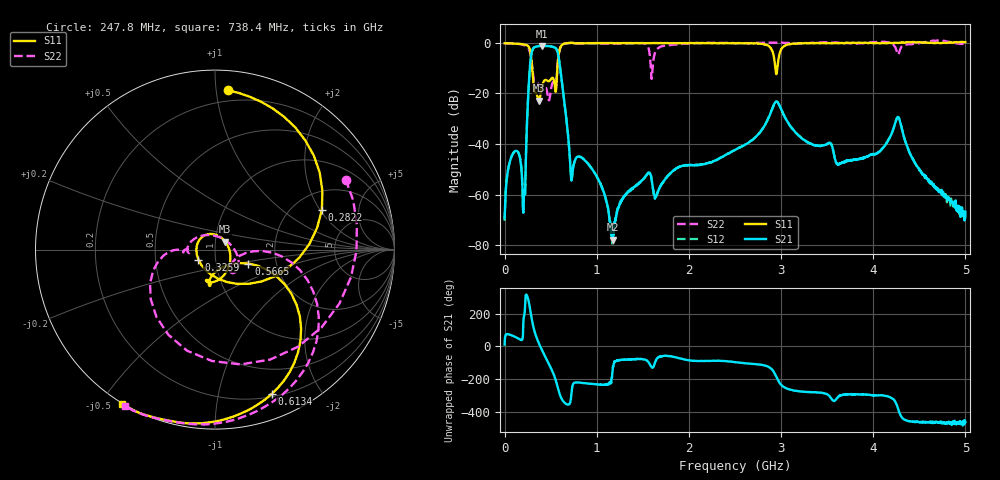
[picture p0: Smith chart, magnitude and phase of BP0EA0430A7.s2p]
!Agilent Technologies,E8358A,US41080443,A.07.50.56
!Agilent E8358A: A.07.50.56
!Date: Friday, November 10, 2017 09:13:59
!Correction: S11(Full 2 Port(1,2))
!S21(Full 2 Port(1,2))
!S12(Full 2 Port(1,2))
!S22(Full 2 Port(1,2))
!S2P File: Measurements: S11, S21, S12, S22:
# Hz S  dB  R 50
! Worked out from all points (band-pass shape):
!   1601 points, 1 MHz to 5 GHz, reference 50 ohm
!   highest |S21| = -1.17 dB at 410.3 MHz (marker M1); lowest = -77.8 dB at 1.173 GHz (marker M2)
!   |S21| within 3 dB of the highest: 292.9 MHz to 579.1 MHz (286.2 MHz wide, 65.7 % of centre)
!   lowest |S11| = -22.8 dB at 372.8 MHz (marker M3), VSWR 1.16, Z = 55.9 + j4.98 ohm
!   |S11| at or under -10 dB: 300.8 MHz to 573.1 MHz (272.3 MHz wide, 62.3 % of centre); 2.939 GHz to 2.96 GHz (21.16 MHz wide, 0.718 % of centre)
!   |S22| runs from -22.7 to 1.0 dB; largest |S21 - S12| = 0.0048
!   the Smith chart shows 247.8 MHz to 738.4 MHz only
!   S11 on the Smith chart (normalised r, x): 247.8 MHz: 0.13, +1.08; 282.2 MHz: 2.79, +2.09; 325.9 MHz: 0.83, -0.09; 566.5 MHz: 1.44, -0.23; 613.4 MHz: 0.23, -1.44; 738.4 MHz: -0.00, -0.57
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1000000  -0.12 179.8  -69.41 10.8  -70.35 12.4  -0.13 179.8
1.041044e8  -0.23 157.3  -43.13 60.1  -43.06 60.2  -0.28 152.1
2.072088e8  -0.57 119.1  -62.78 169.5  -62.49 171.2  -0.78 96.3
2.478256e8  -1.01 85.3  -28.08 -55.9  -28.04 -55.9  -1.66 28.2
2.821938e8  -3.93 20.5  -6.92 -149.1  -6.88 -149.1  -4.66 -105.4
3.25935e8  -19.34 -148.9  -1.70 90.4  -1.65 90.4  -15.05 -175.7
3.728006e8  -22.79 37.7  -1.25 17.7  -1.21 17.7  -16.58 -179.5
4.102931e8  -16.69 -67.8  -1.17 -28.0  -1.14 -27.9  -16.48 -173.7
4.821538e8  -15.16 -103.3  -1.26 -107.9  -1.22 -107.9  -22.69 66.9
5.665119e8  -13.89 -22.6  -2.69 131.7  -2.65 131.7  -13.43 -2.5
6.133775e8  -1.27 -68.6  -12.68 45.7  -12.64 45.8  -1.33 -57.9
7.383525e8  0.03 -121.0  -51.05 121.0  -50.94 121.2  0.05 -119.8
8.352081e8  -0.13 -135.1  -45.27 136.2  -45.29 136.8  -0.15 -133.3
1.172641e9  -0.06 -156.5  -77.81 -155.7  -80.38 -135.3  -0.23 -167.6
1.572561e9  -0.07 -167.9  -51.31 -106.1  -51.11 -106.0  -3.86 172.7
1.669416e9  -0.08 -169.5  -58.49 -67.8  -58.08 -66.1  -1.98 -109.4
2.5005e9  -0.15 171.0  -42.36 -97.3  -42.30 -97.1  -0.12 -179.3
2.944161e9  -11.69 19.4  -23.24 178.4  -23.19 178.4  0.12 176.3
3.059763e9  -0.75 -161.1  -30.54 102.3  -30.52 102.9  0.04 170.9
3.334708e9  -0.07 173.4  -40.02 79.0  -40.03 79.5  0.05 161.8
4.168916e9  0.01 156.6  -38.13 51.3  -38.12 51.9  0.18 153.4
5e9  0.33 150.2  -66.71 -103.5  -67.69 -116.6  -0.45 156.0
